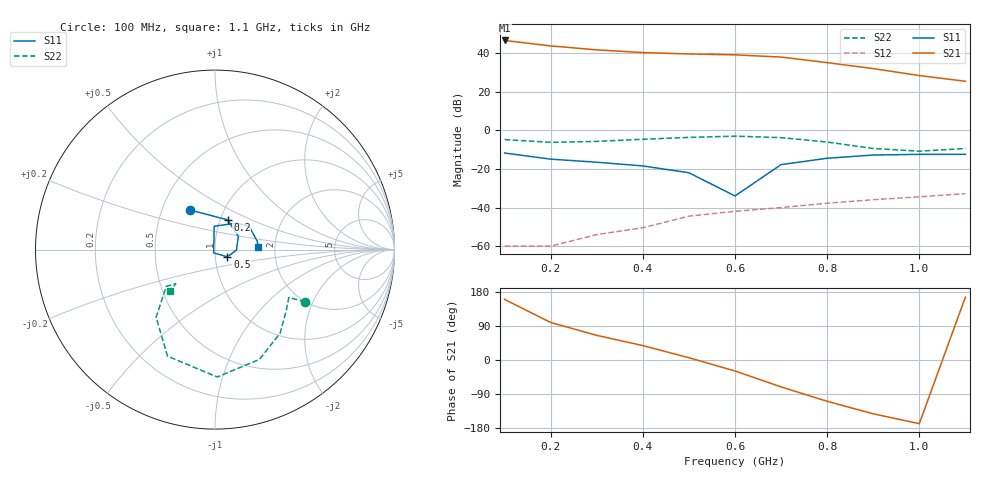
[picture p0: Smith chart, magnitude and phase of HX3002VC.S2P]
!  HPMX-3002  S PARAMETERS
!  Vcc1=4.5 V, Vcc2=6 V, Vcontrol = 1.6 V
!  LAST UPDATED 01 07 94
# ghz s ma r 50
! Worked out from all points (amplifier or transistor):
!   11 points, 100 MHz to 1.1 GHz, reference 50 ohm
!   highest |S21| = 46.6 dB at 100 MHz (marker M1)
!   |S21| within 3 dB of that: start of sweep to 208.1 MHz
!   unconditionally stable (mu >= 1): start of sweep to 440.4 MHz; 910.3 MHz to end of sweep
!   at 200 MHz: K = 2.53, MAG = 45.0 dB, |S12| = -60.0 dB
!   at 600 MHz: K = 0.69, MSG = 40.6 dB, |S12| = -41.9 dB
!   at 1.1 GHz: K = 1.15, MAG = 26.8 dB, |S12| = -32.8 dB
!   S11 on the Smith chart (normalised r, x): 100 MHz: 0.69, +0.33; 200 MHz: 1.09, +0.37; 500 MHz: 1.14, -0.09; 1.1 GHz: 1.63, +0.06
0.1  0.26 122.0  214.7 160.0  0.001 111.0  0.58 -30.0
0.2  0.18 67.0  154.9 99.0  0.001 133.0  0.49 -33.0
0.3  0.15 30.0  122.5 65.0  0.002 139.0  0.52 -40.0
0.4  0.12 -1.0  104.2 38.0  0.003 149.0  0.59 -52.0
0.5  0.08 -30.0  95.89 6.0  0.006 148.0  0.66 -68.0
0.6  0.02 -112.0  90.91 -29.0  0.008 142.0  0.71 -89.0
0.7  0.13 92.0  79.7 -71.0  0.01 137.0  0.65 -114.0
0.8  0.19 51.0  57.23 -109.0  0.013 135.0  0.5 -131.0
0.9  0.23 34.0  39.99 -142.0  0.016 134.0  0.34 -143.0
1  0.24 11.0  26.42 -168.0  0.019 132.0  0.29 -139.0
1.1  0.24 4.0  18.82 166.0  0.023 129.0  0.34 -137.0
